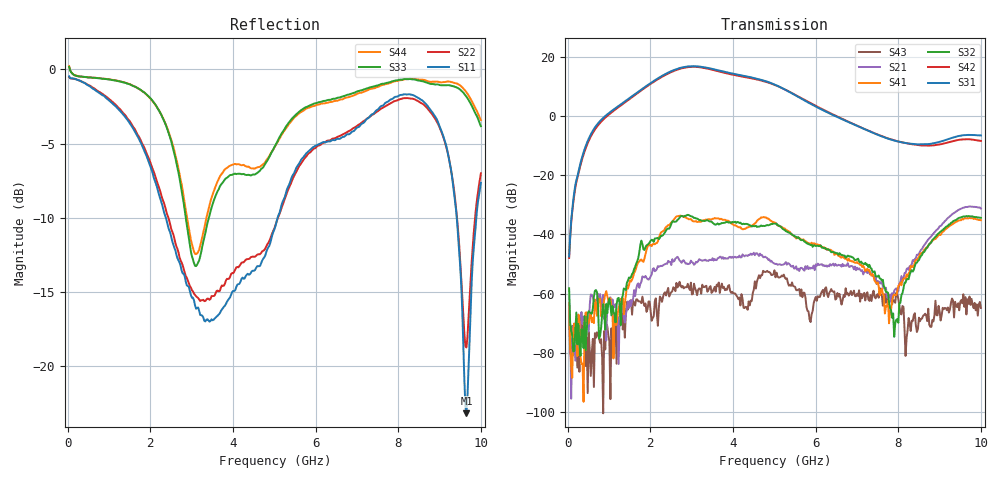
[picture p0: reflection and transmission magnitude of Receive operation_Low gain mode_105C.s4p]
! Device:  ADRF5545A
! Description: Dual-Channel, Receiver Front End
! Frequency:  2.4 -  4.2 GHz
! Ports:
!	ANT-CHA	= Port 1
!	ANT-CHB	= Port 2
!  RXOUT-CHA = Port 3
!	RXOUT-CHB = Port 4
! VDD1-CHA, VDD1-CHB, VDD2-CHA, VDD2-CHB, and SWVDD-CHAB = 5 V
! SWCTRL-CHAB = 0 V,  PD-CHAB = 0 V,BP-CHA=BP-CHB=5V
! Temp=105C
! Data:  Data was collected using a calibrated 4 port network analyzer and de-embedded using AtaiTec's In Situ De-Embedding.
! Note:  Analog Devices supplies this data as a sample of measured data
!  for this product.  Your particular data for this product may vary.
!  Data was taken at 105 degrees C.
!  Analog Devices reserves the right to change this data at anytime.
!Correction: S11(Full 4 Port(1,2,3,4))
!S12(Full 4 Port(1,2,3,4))
!S13(Full 4 Port(1,2,3,4))
!S14(Full 4 Port(1,2,3,4))
!S21(Full 4 Port(1,2,3,4))
!S22(Full 4 Port(1,2,3,4))
!S23(Full 4 Port(1,2,3,4))
!S24(Full 4 Port(1,2,3,4))
!S31(Full 4 Port(1,2,3,4))
!S32(Full 4 Port(1,2,3,4))
!S33(Full 4 Port(1,2,3,4))
!S34(Full 4 Port(1,2,3,4))
!S41(Full 4 Port(1,2,3,4))
!S42(Full 4 Port(1,2,3,4))
!S43(Full 4 Port(1,2,3,4))
!S44(Full 4 Port(1,2,3,4))
!S4P File: Measurements: <S11,S12,S13,S14>,
!<S21,S22,S23,S24>,
!<S31,S32,S33,S34>,
!<S41,S42,S43,S44>:
# Hz S  dB  R 50
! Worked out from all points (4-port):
!   400 points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, 34.98 MHz to 10 GHz, reference 50 ohm
!   strongest paths, dB at 34.98 MHz, 2.532 GHz, 5.03 GHz, 7.527 GHz, 10 GHz:
!     S31: -47.4, 15.4, 10.6, -6.4, -6.5
!     S42: -47.9, 15.1, 10.5, -6.4, -8.4
!     S32: -58.2, -35.6, -36.3, -53.9, -34.4
!     S41: -63.3, -35.7, -36.1, -57.6, -35.2
!     S21: -63.5, -48.4, -50.0, -55.9, -31.2
!     S43: -66.7, -59.2, -54.5, -61.4, -64.9
!   lowest |S11| = -23.2 dB at 9.65 GHz (marker M1), VSWR 1.15, Z = 44.5 + j3.53 ohm
!   |S11| at or under -10 dB: 2.378 GHz to 5.079 GHz (2.701 GHz wide, 72.5 % of centre); 9.416 GHz to 9.89 GHz (474.2 MHz wide, 4.91 % of centre)
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3.4975e7  -0.47 -10.2  -66.15 -106.3  -66.20 -108.3  -69.03 23.3
          -63.46 61.1  -0.52 -10.0  -62.60 -174.6  -59.36 -159.3
          -47.43 -7.2  -58.20 -72.1  0.18 -6.4  -65.55 -59.1
          -63.31 -179.7  -47.95 -6.0  -66.70 -18.8  0.22 -6.3
2.182825e9  -8.16 -158.1  -52.22 100.2  -43.94 116.4  -72.79 151.3
            -50.70 94.1  -7.73 -156.9  -73.23 110.8  -44.48 120.5
            12.78 138.6  -41.17 51.0  -2.64 -103.6  -58.47 151.5
            -42.33 73.7  12.50 141.2  -70.89 174.4  -2.65 -105.1
3.25675e9  -16.58 37.0  -48.80 41.4  -34.48 7.8  -67.31 57.6
           -48.89 37.8  -15.54 39.9  -71.41 38.4  -35.14 10.5
           16.66 8.6  -35.39 -88.0  -11.93 -87.1  -56.96 86.3
           -35.34 -76.7  16.42 11.7  -57.00 83.5  -11.28 -90.8
4.006e9  -14.91 -13.5  -47.67 14.5  -34.00 -56.6  -68.14 34.9
         -47.90 16.8  -13.72 -1.1  -71.26 40.0  -34.62 -51.7
         14.37 -66.4  -35.87 -151.2  -7.06 -103.2  -57.83 36.5
         -36.74 -159.4  14.00 -62.4  -59.91 -11.4  -6.40 -99.4
4.9051e9  -11.67 35.2  -46.75 -8.3  -34.36 -129.3  -70.95 -3.9
          -49.17 -28.7  -11.38 39.1  -72.03 -76.8  -34.67 -123.5
          11.29 -151.3  -36.64 134.1  -5.76 164.7  -67.79 110.6
          -35.30 120.6  11.12 -145.6  -53.02 90.5  -5.71 172.8
9.65035e9  -23.15 145.4  -31.20 -124.0  -42.62 51.4  -58.29 67.5
           -30.72 -124.7  -18.72 149.1  -61.42 64.9  -43.38 60.2
           -6.36 -33.0  -33.79 -96.1  -1.83 94.5  -63.02 23.9
           -34.58 -94.9  -7.81 -29.5  -67.06 12.0  -1.54 91.1
1e10  -7.64 -148.7  -31.48 -178.6  -42.61 30.6  -55.44 47.3
      -31.20 179.0  -7.00 -156.8  -59.88 32.9  -44.70 29.5
      -6.53 -69.2  -34.40 -155.3  -3.82 91.6  -60.68 10.5
      -35.22 -155.3  -8.38 -64.1  -64.86 27.1  -3.41 90.4
